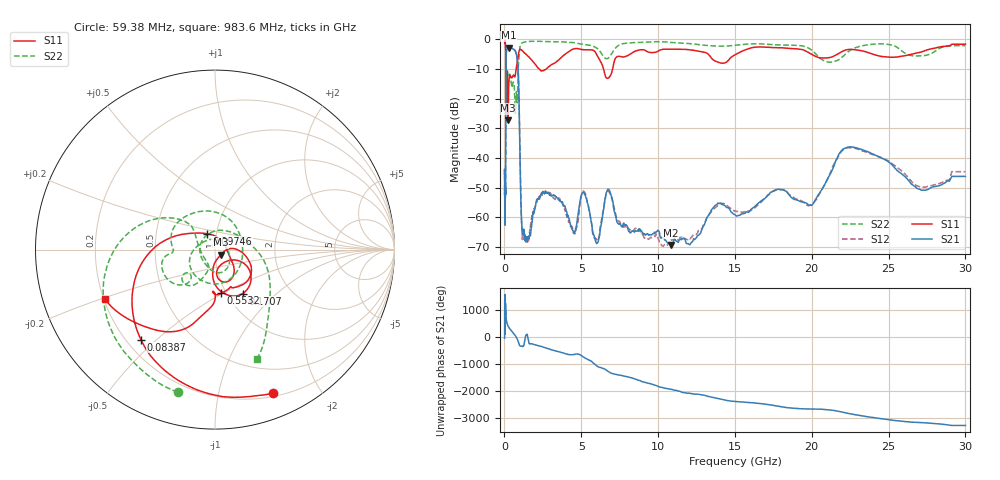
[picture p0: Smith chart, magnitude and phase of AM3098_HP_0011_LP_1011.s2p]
! Date/Time: Thu, Feb 28, 2019 8:34 AM
! Network Analyzer: Agilent Technologies E8364B Rev: A.07.50.67
! Sweep from 0.010 to 30.000 GHz, 1601 Points, Sweep Type: LOG
! Power Supply: 5.022 V, 0.002 A
# Hz S DB R 50
!freq MagS11 AngS11 MagS21 AngS21 MagS12 AngS12 MagS22 AngS22
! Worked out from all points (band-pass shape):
!   1601 points, 10 MHz to 30 GHz, reference 50 ohm
!   highest |S21| = -2.82 dB at 271.8 MHz (marker M1); lowest = -69.3 dB at 10.81 GHz (marker M2)
!   |S21| within 3 dB of the highest: 108.7 MHz to 807.3 MHz (698.6 MHz wide, 153 % of centre)
!   lowest |S11| = -27.2 dB at 233.9 MHz (marker M3), VSWR 1.09, Z = 53.3 - j3.08 ohm
!   |S11| at or under -10 dB: 93.01 MHz to 756.6 MHz (663.6 MHz wide, 156 % of centre); 2.269 GHz to 2.711 GHz (442.3 MHz wide, 17.8 % of centre); 6.451 GHz to 7.037 GHz (586.2 MHz wide, 8.69 % of centre)
!   |S22| runs from -24.9 to -0.6 dB; largest |S21 - S12| = 0.013
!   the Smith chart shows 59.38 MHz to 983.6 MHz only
!   S11 on the Smith chart (normalised r, x): 59.38 MHz: 0.23, -1.46; 83.87 MHz: 0.26, -0.45; 97.46 MHz: 0.90, +0.16; 170.7 MHz: 1.18, -0.63; 553.2 MHz: 0.94, -0.49; 983.6 MHz: 0.21, -0.21
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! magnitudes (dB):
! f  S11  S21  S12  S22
! 10 MHz  -0.3  -45.5  -44.1  -0.6
! 38.04 MHz  -0.5  -61.1  -59.8  -1.0
! 59.38 MHz  -1.3  -53.1  -53.2  -1.7
! 83.87 MHz  -3.7  -34.9  -35.0  -4.2
! 97.46 MHz  -19.9  -10.8  -10.8  -21.8
! 144.7 MHz  -15.4  -3.6  -3.5  -13.2
! 170.7 MHz  -10.8  -3.4  -3.4  -10.1
! 233.9 MHz  -27.2  -2.9  -2.9  -12.4
! 271.8 MHz  -16.5  -2.8  -2.8  -12.6
! 550.5 MHz  -12.2  -3.2  -3.2  -14.6
! 553.2 MHz  -12.2  -3.2  -3.2  -14.5
! 850.8 MHz  -6.6  -7.6  -7.6  -19.1
! 983.6 MHz  -3.5  -31.1  -31.0  -3.7
! 1.196 GHz  -4.0  -64.7  -66.1  -1.0
! 2.084 GHz  -8.9  -54.3  -54.9  -0.6
! 5.989 GHz  -4.9  -68.8  -67.4  -2.9
! 6.787 GHz  -12.9  -50.5  -51.1  -6.2
! 7.926 GHz  -5.7  -62.5  -62.9  -1.3
! 10.81 GHz  -3.3  -69.3  -68.3  -1.0
! 19.8 GHz  -4.5  -55.9  -56.1  -2.9
! 22.67 GHz  -3.4  -36.3  -36.5  -3.2
! 30 GHz  -1.6  -46.2  -44.6  -2.1
